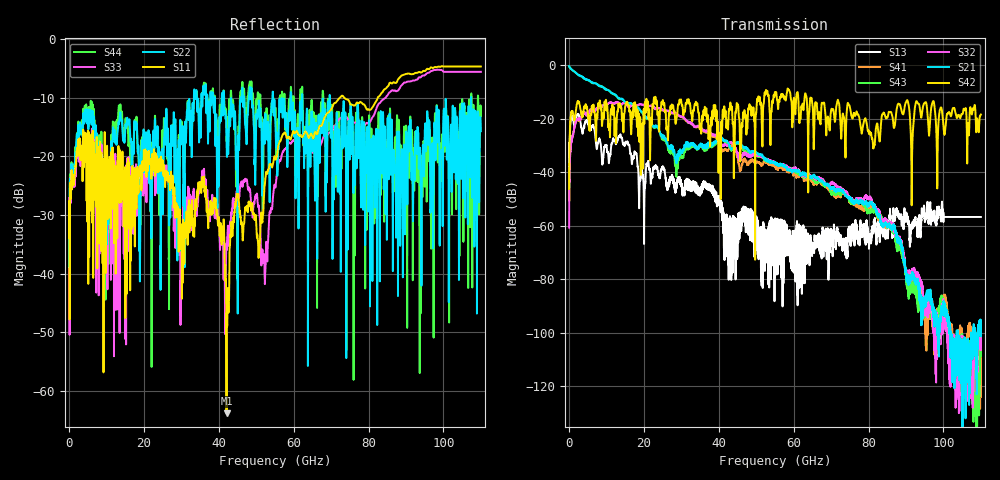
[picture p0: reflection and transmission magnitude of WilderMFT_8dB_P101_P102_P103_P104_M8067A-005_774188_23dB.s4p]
# GHz S RI R 50
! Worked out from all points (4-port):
!   11000 points, 10 MHz to 110 GHz, reference 50 ohm
!   strongest paths, dB at 10 MHz, 27.51 GHz, 55.01 GHz, 82.51 GHz, 110 GHz:
!     S42: -46.2, -15.0, -9.9, -23.8, -18.4
!     S21: -0.3, -31.3, -36.8, -55.4, -101.0
!     S32: -60.7, -17.6, -36.4, -54.2, -106.6
!     S43: -0.4, -32.4, -36.5, -56.6, -107.8
!     S41: -42.4, -17.9, -38.1, -56.8, -124.2
!     S13: -29.1, -41.3, -58.9, -57.6, -56.7
!   lowest |S11| = -63.8 dB at 42.06 GHz (marker M1), VSWR 1.00, Z = 50 - j0.0647 ohm
!   |S11| at or under -10 dB: start of sweep to 72.4 GHz; 73.45 GHz to 82.49 GHz (9.034 GHz wide, 11.6 % of centre)
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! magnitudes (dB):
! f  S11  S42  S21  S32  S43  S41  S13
! 10 MHz  -33.9  -46.2  -0.3  -60.7  -0.4  -42.4  -29.1
! 1.91 GHz  -20.0  -15.7  -2.9  -20.8  -2.8  -20.8  -19.8
! 10.86 GHz  -20.7  -23.9  -9.7  -14.0  -9.7  -14.1  -33.8
! 28.66 GHz  -28.1  -20.2  -36.3  -17.8  -41.0  -18.0  -45.2
! 42.06 GHz  -63.8  -23.1  -28.3  -29.9  -28.8  -31.7  -61.1
! 57.29 GHz  -16.2  -11.5  -37.5  -37.3  -37.3  -38.4  -66.7
! 110 GHz  -4.7  -18.4  -101.0  -106.6  -107.8  -124.2  -56.7
